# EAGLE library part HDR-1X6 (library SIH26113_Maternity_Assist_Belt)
1x6 2.54 mm pin header
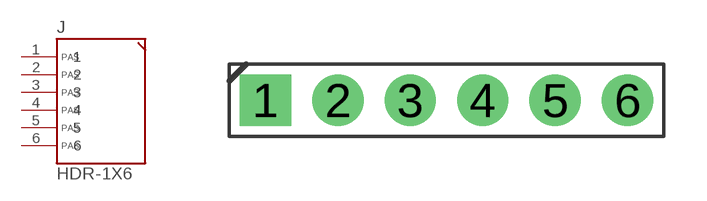
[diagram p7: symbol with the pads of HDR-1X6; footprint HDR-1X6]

Designator prefix J

## HDR-1X6  [HDR-1X6]
1  1  pas
2  2  pas
3  3  pas
4  4  pas
5  5  pas
6  6  pas

## Footprint HDR-1X6 (pad centres in mm)
1x6 2.54 mm through-hole pin header. Drill 1.0 mm / pad 1.8 mm suits the 0.64 mm square posts used by all common 2.54 mm headers. Pad 1 is square.
drill 1 pad 1.8 square: 1 -6.35,0
drill 1 pad 1.8: 2 -3.81,0; 3 -1.27,0; 4 1.27,0; 5 3.81,0; 6 6.35,0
